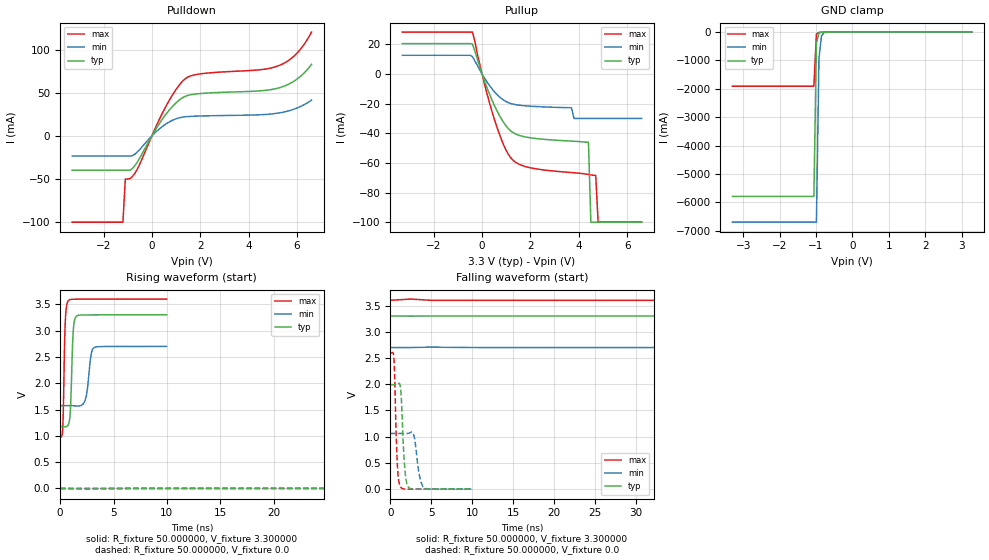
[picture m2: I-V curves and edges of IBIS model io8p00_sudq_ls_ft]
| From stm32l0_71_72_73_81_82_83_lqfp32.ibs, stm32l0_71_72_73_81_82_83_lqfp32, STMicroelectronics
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|   Model io8p00_sudq_ls_ft
[Model]  io8p00_sudq_ls_ft
Model_type I/O
Polarity   Non-Inverting
Enable   Active-Low
Vinl =   0.990000V
Vinh =   2.310000V
Vmeas =  1.650000V
Cref =   50.000000pF
Rref =   100.000000M
Vref =   0.0V
C_comp   2.343000pF   2.309800pF   2.393900pF
[Temperature Range]   25.000000   0.125000k   -40.000000
[Pullup Reference]   3.300000V   2.700000V   3.600000V
[Pulldown Reference]   0.0V   0.0V   0.0V
[POWER Clamp Reference]   3.300000V   2.700000V   3.600000V
[GND Clamp Reference]   0.0V   0.0V   0.0V
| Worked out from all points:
|   slope of the pulldown table from 0 to 0.495 V, typ, clamps not added: 22.6 ohm
|   slope of the pullup table from 0 to 0.495 V, typ, clamps not added: 23.9 ohm
|   GND clamp passes 1 mA (typ) near -0.64 V on its own axis
|   rising waveform, R_fixture 50.000000, V_fixture 3.300000: 20-80 % time 208ps typ, 362ps min, 165ps max; typ from 1.18 V to 3.3 V
|   rising waveform, R_fixture 50.000000, V_fixture 0.0: 20-80 % time 205ns typ, 426ns min, 99.7ns max; typ from 0 V to 1.99 V
|   falling waveform, R_fixture 50.000000, V_fixture 3.300000: 20-80 % time 193ns typ, 383ns min, 106ns max; typ from 3.3 V to 1.18 V
|   falling waveform, R_fixture 50.000000, V_fixture 0.0: 20-80 % time 380ps typ, 552ps min, 301ps max; typ from 1.99 V to 0 V
[Pulldown]
|Voltage   I(typ)   I(min)   I(max)
-3.3V     -39.8mA    -23.37mA   -100mA
-1.2V     -39.8mA    -23.37mA   -100mA
-1.1V     -39.8mA    -23.37mA   -50.1mA
-900mV    -39.8mA    -23.37mA   -49.43mA
-700mV    -34.25mA   -21mA      -43.13mA
600mV     25.84mA    14.18mA    35.34mA
1V        38.32mA    19.82mA    53.81mA
1.4V      46.09mA    22.19mA    66.63mA
2V        49.05mA    23.02mA    71.83mA
5.2V      55.23mA    26.32mA    80.92mA
6V        65.76mA    32.26mA    95.84mA
6.6V      82.81mA    41.43mA    120.2mA
[Pullup]
|Voltage   I(typ)   I(min)   I(max)
-3.3V     20.52mA    12.64mA    28.28mA
-400mV    20.25mA    11.77mA    28.28mA
500mV     -20.88mA   -11.78mA   -30.07mA
1.2V      -38.62mA   -19.99mA   -56.79mA
1.9V      -42.79mA   -21.61mA   -62.92mA
3.7V      -45.29mA   -22.8mA    -66.5mA
3.8V      -45.39mA   -30mA      -66.64mA
4.4V      -46mA      -30mA      -67.77mA
4.5V      -100mA     -30mA      -68.06mA
4.7V      -100mA     -30mA      -68.4mA
4.8V      -100mA     -30mA      -100mA
6.6V      -100mA     -30mA      -100mA
[GND_clamp]
|Voltage   I(typ)   I(min)   I(max)
-3.3V     -5.787A    -6.696A    -1.906A
-1.06V    -5.787A    -6.696A    -1.906A
-990mV    -393.4mA   -6.696A    -70.75mA
-920mV    -33.02mA   -919.4mA   -10.9mA
-850mV    -6.829mA   -131.3mA   -6.521mA
-780mV    -3.478mA   -21.06mA   -4.208mA
3.28V     0A         0A         0A
[POWER_clamp]
|Voltage   I(typ)   I(min)   I(max)
-3.28V    0A         0A         0A
0V        0A         0A         0A
[Ramp]
| variable   typ   min   max
dV/dt_r  1.19496/0.20440u   0.61230/0.42777u   1.55568/99.58129n
dV/dt_f  1.27272/0.19288u   0.63564/0.38274u   1.57787/0.10598u
R_load = 50.000000
[Rising Waveform]
R_fixture= 50.000000
V_fixture= 3.300000
V_fixture_min= 2.700000
V_fixture_max= 3.600000
|time   V(typ)   V(min)   V(max)
0s        1.177V     1.573V     968.3mV
240.2ps   1.176V     1.573V     1.137V
480.5ps   1.173V     1.573V     3.169V
760.8ps   1.214V     1.573V     3.569V
961ps     1.499V     1.573V     3.592V
1.221ns   2.977V     1.572V     3.596V
1.502ns   3.269V     1.569V     3.597V
2.382ns   3.298V     1.702V     3.599V
3.203ns   3.299V     2.679V     3.599V
9.97ns    3.3V       2.7V       3.6V
[Rising Waveform]
R_fixture= 50.000000
V_fixture= 0.0
V_fixture_min= 0.0
V_fixture_max= 0.0
|time   V(typ)   V(min)   V(max)
0s        2.053nV    14.4nV     4.46nV
50.05ns   269.3uV    -22.04uV   84.31mV
102.6ns   83.68mV    140.9uV    950.7mV
162.7ns   432.5mV    2.564mV    1.898V
202.7ns   722.6mV    16.04mV    2.272V
250.2ns   1.051V     48.7mV     2.472V
355.4ns   1.572V     183.4mV    2.572V
495.5ns   1.87V      425.2mV    2.59V
818.3ns   1.985V     867.9mV    2.592V
1.246us   1.992V     1.062V     2.592V
[Falling Waveform]
R_fixture= 50.000000
V_fixture= 3.300000
V_fixture_min= 2.700000
V_fixture_max= 3.600000
|time   V(typ)   V(min)   V(max)
0s        3.3V       2.7V       3.6V
82.58ns   3.3V       2.7V       3.497V
145.1ns   3.215V     2.7V       2.593V
217.7ns   2.819V     2.696V     1.543V
255.3ns   2.561V     2.685V     1.202V
292.8ns   2.293V     2.662V     1.073V
407.9ns   1.573V     2.532V     993mV
520.5ns   1.312V     2.339V     976.4mV
878.4ns   1.191V     1.743V     968.7mV
1.246us   1.177V     1.573V     968.3mV
[Falling Waveform]
R_fixture= 50.000000
V_fixture= 0.0
V_fixture_min= 0.0
V_fixture_max= 0.0
|time   V(typ)   V(min)   V(max)
0s        1.992V     1.062V     2.592V
440.4ps   1.992V     1.062V     2.506V
860.9ps   1.996V     1.062V     482.1mV
1.261ns   1.916V     1.062V     39.71mV
1.762ns   425.2mV    1.061V     3.009mV
2.222ns   38.19mV    1.065V     1.16mV
2.883ns   1.939mV    1.025V     742.8uV
3.524ns   657.4uV    293mV      502.1uV
4.024ns   437uV      43.02mV    375.5uV
9.97ns    2.053nV    14.4nV     4.46nV
